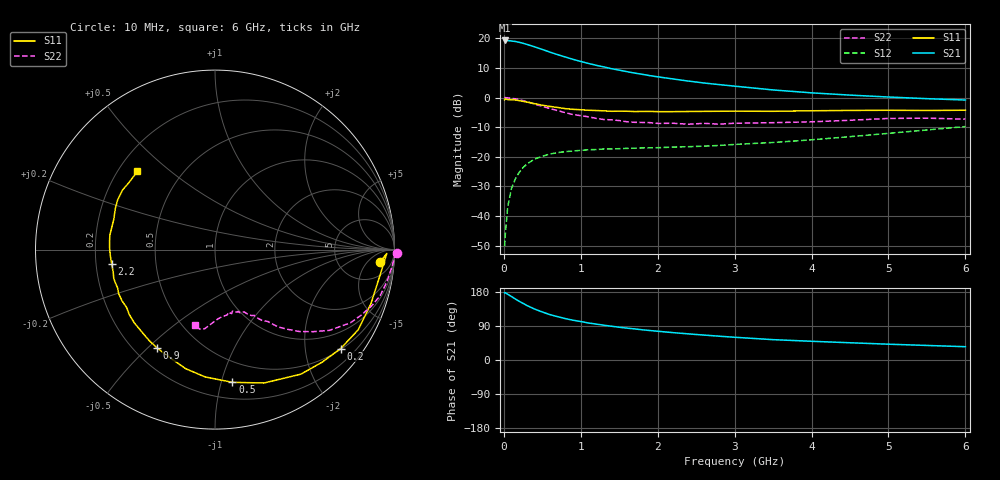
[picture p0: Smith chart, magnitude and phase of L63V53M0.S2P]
!  INFINEON TECHNOLOGIES Small Signal Semiconductors
! BFR380L3 , Si-NPN RF-Transistor in TSLP-3-1
!  Vce=3.5 V,  Ic=3 mA
! Common Emitter S-Parameters:  07. March 2005
#  GHz  S  MA  R  50
! f  S11  S21  S12  S22
! GHz  Mag  Ang  Mag  Ang  Mag  Ang  Mag  Ang
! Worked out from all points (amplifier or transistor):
!   36 points, 10 MHz to 6 GHz, reference 50 ohm
!   highest |S21| = 19.3 dB at 10 MHz (marker M1)
!   |S21| within 3 dB of that: start of sweep to 495.4 MHz
!   unconditionally stable (mu >= 1): 2.714 GHz to 4.627 GHz
!   at 250 MHz: K = 0.11, MSG = 21.0 dB, |S12| = -23.6 dB
!   at 1.4 GHz: K = 0.63, MSG = 13.6 dB, |S12| = -17.3 dB
!   at 6 GHz: K = 0.90, MSG = 4.5 dB, |S12| = -9.8 dB
!   S11 on the Smith chart (normalised r, x): 10 MHz: 13, -12; 200 MHz: 0.52, -2.80; 500 MHz: 0.33, -1.09; 900 MHz: 0.29, -0.53; 2.2 GHz: 0.27, -0.06; 6 GHz: 0.28, +0.39
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0.01  0.9203 -4.4  9.262 177.0  0.0031 89.6  1.014 -1.1
0.02  0.9573 -1.3  9.241 177.7  0.0051 93.3  1.001 -2.3
0.05  0.9281 -9.9  9.22 173.5  0.0142 86.2  0.9917 -5.3
0.1  0.9195 -19.2  9.063 167.3  0.0295 80.2  0.9748 -10.5
0.15  0.9146 -29.2  8.904 161.0  0.0426 74.0  0.9553 -15.6
0.2  0.8912 -38.2  8.615 154.8  0.0547 70.3  0.9267 -19.9
0.3  0.843 -55.4  7.934 143.8  0.0757 61.7  0.8575 -28.4
0.4  0.7919 -69.8  7.233 134.4  0.0919 54.7  0.7805 -35.2
0.5  0.7459 -82.5  6.526 126.7  0.1025 49.6  0.7128 -39.9
0.6  0.7116 -94.4  5.879 119.7  0.1118 45.3  0.6548 -44.2
0.7  0.6834 -103.8  5.327 114.3  0.118 42.3  0.6031 -47.5
0.8  0.6532 -112.3  4.861 109.2  0.1226 39.9  0.5589 -50.6
0.9  0.636 -120.5  4.44 105.0  0.1256 38.1  0.519 -52.6
1.1  0.6128 -132.3  3.79 97.7  0.1319 36.1  0.4746 -56.4
1.3  0.5991 -142.9  3.309 91.8  0.1359 35.2  0.4271 -59.2
1.6  0.59 -155.6  2.753 84.1  0.1392 35.4  0.3915 -64.2
2.2  0.581 -172.1  2.071 72.2  0.1463 39.2  0.37 -70.5
2.8  0.5895 175.0  1.662 62.8  0.1559 45.2  0.3574 -78.2
3.5  0.5887 163.3  1.351 53.7  0.1751 51.4  0.3783 -85.0
4.5  0.6089 153.0  1.105 45.5  0.2196 60.3  0.4152 -93.1
5.5  0.6078 141.4  0.962 38.4  0.2849 63.4  0.4508 -101.1
6  0.6141 134.7  0.913 35.1  0.3249 63.1  0.434 -105.1
